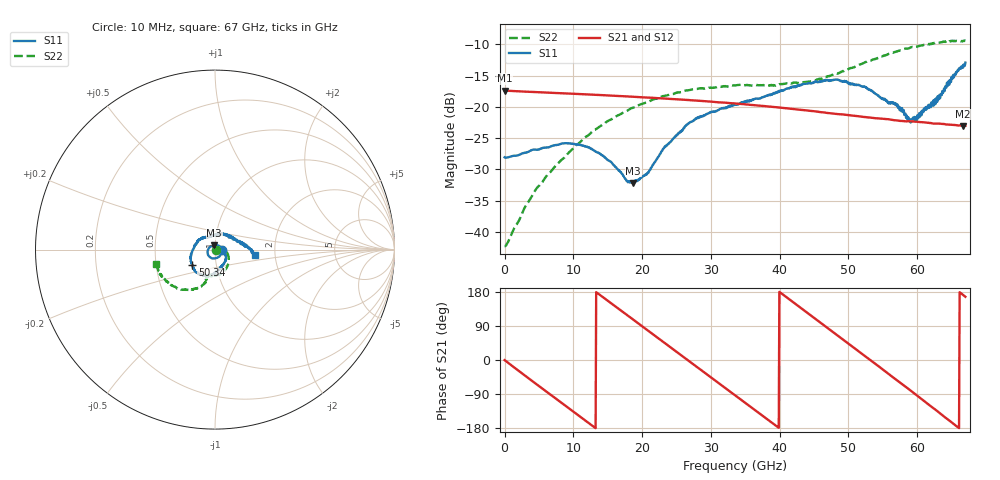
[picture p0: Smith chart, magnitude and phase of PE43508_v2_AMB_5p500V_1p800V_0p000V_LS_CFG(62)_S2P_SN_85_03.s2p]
!Keysight Technologies,N5227A,US51270237,A.10.43.00
!Date: Wednesday, August 22, 2018 17:13:04
!Correction: S11(Full 2 Port(1,3))
!S31(Full 2 Port(1,3))
!S13(Full 2 Port(1,3))
!S33(Full 2 Port(1,3))
!S2P File: Measurements: S11, S31, S13, S33:
# Hz S  dB  R 50
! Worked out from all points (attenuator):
!   801 points, 10 MHz to 67 GHz, reference 50 ohm
!   highest |S21| = -17.39 dB at 10 MHz (marker M1); lowest = -23.0 dB at 66.67 GHz (marker M2)
!   lowest |S11| = -32.2 dB at 18.68 GHz (marker M3), VSWR 1.05, Z = 49.5 + j2.4 ohm
!   |S11| at or under -10 dB: start of sweep to end of sweep
!   |S22| runs from -42.2 to -9.4 dB; largest |S21 - S12| = 0.00071
!   S11 on the Smith chart (normalised r, x): 10 MHz: 1.08, -0.00; 50.34 GHz: 0.76, -0.14; 67 GHz: 1.57, -0.10
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1e7  -28.06 -0.8  -17.39 -0.2  -17.39 -0.2  -42.23 -1.0
4.615562e9  -26.86 -61.5  -17.65 -63.5  -17.65 -63.5  -33.09 27.8
7.797588e9  -26.06 -99.9  -17.81 -106.6  -17.80 -106.5  -29.02 17.3
1.123082e10  -26.14 -136.4  -17.97 -152.9  -17.98 -152.8  -25.36 -0.9
1.466406e10  -28.12 -177.0  -18.16 160.9  -18.15 161.0  -22.52 -18.8
1.784609e10  -31.81 123.0  -18.33 118.2  -18.33 118.2  -20.61 -34.8
1.868346e10  -32.15 100.7  -18.38 106.9  -18.38 106.9  -20.14 -38.3
2.07769e10  -30.56 47.9  -18.52 78.7  -18.51 78.7  -19.23 -48.5
2.236791e10  -27.95 14.4  -18.62 57.3  -18.61 57.3  -18.59 -55.8
2.6806e10  -22.62 -34.0  -18.91 -2.4  -18.91 -2.4  -17.34 -73.2
3.040671e10  -20.81 -57.0  -19.20 -51.0  -19.19 -51.0  -16.93 -85.2
3.3505e10  -19.65 -72.1  -19.47 -92.9  -19.47 -92.9  -16.58 -93.8
3.919915e10  -17.76 -89.6  -20.02 -169.9  -20.02 -169.8  -16.56 -101.9
4.472582e10  -16.18 -112.7  -20.65 115.0  -20.64 115.1  -15.90 -105.5
4.815906e10  -15.64 -131.4  -21.12 68.3  -21.12 68.2  -14.76 -106.4
5.033624e10  -16.25 -145.2  -21.38 38.6  -21.37 38.6  -13.79 -108.1
5.251341e10  -16.92 -162.5  -21.64 8.7  -21.62 8.7  -12.82 -112.4
5.586291e10  -19.47 159.8  -21.98 -37.3  -21.97 -37.6  -11.52 -122.3
5.937989e10  -21.71 100.6  -22.33 -85.3  -22.34 -85.5  -10.43 -133.9
6.29806e10  -18.29 35.6  -22.65 -135.9  -22.67 -136.3  -9.80 -148.7
6.666505e10  -13.73 -4.9  -23.04 171.7  -23.10 171.8  -9.46 -164.1
6.7e10  -12.94 -8.0  -23.02 166.8  -23.09 166.9  -9.43 -166.0
